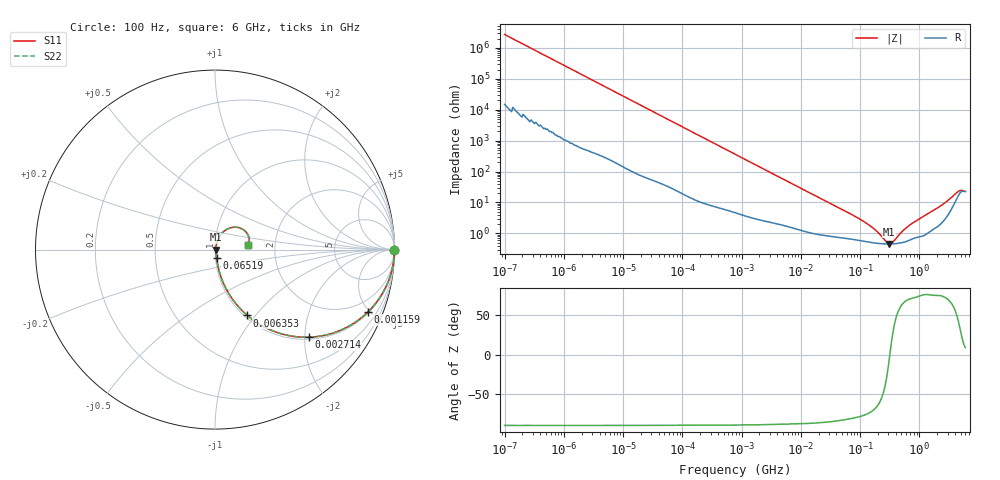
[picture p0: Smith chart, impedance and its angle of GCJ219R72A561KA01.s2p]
!Murata Part Number: GCJ219R72A561KA01
!These Parameters are Measured in Series Mode Connection
!Data Generated on Mar 13, 2026
!  o--ll--o
!Port1  Port2
!  o------o
!Operation Temp=25[degC], DC Bias Voltage=0[V]
!Freq. Start=100[Hz] Stop=6[GHz] 401[Steps]
# Hz S RI R 50
!Freq.(Hz) S11(Real) S11(Imag) S21(Real) S21(Imag) S12(Real) S12(Imag) S22(Real) S22(Imag)
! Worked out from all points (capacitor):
!   401 points, 100 Hz to 6 GHz, reference 50 ohm
!   read as one part in series: C = 580 pF near 109 Hz
!   lowest |Z| = 456 mohm at 312.4 MHz (marker M1)
!   series resonance near 318.1 MHz, so ESL is about 430 pH
!   S11 on the Smith chart (normalised r, x): 100 Hz: open; 1.159 MHz: 1.07, -4.88; 2.714 MHz: 1.05, -2.10; 6.353 MHz: 1.03, -0.91; 65.19 MHz: 1.01, -0.09; 6 GHz: 1.45, +0.07
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100  1 -3.65e-05  2e-07 3.65e-05  2e-07 3.65e-05  1 -3.65e-05
280  1 -0.000102  5e-07 0.000102  5e-07 0.000102  1 -0.000102
2008  1 -0.000728  3.5e-06 0.000728  3.5e-06 0.000728  1 -0.000728
40335  0.9997 -0.0145  0.0003 0.0145  0.0003 0.0145  0.9997 -0.0145
231233  0.9926 -0.0818  0.00737 0.0818  0.00737 0.0818  0.9926 -0.0818
774597  0.9272 -0.2535  0.0728 0.2535  0.0728 0.2535  0.9272 -0.2535
1159002  0.8528 -0.347  0.1472 0.347  0.1472 0.347  0.8528 -0.347
2713602  0.524 -0.4882  0.476 0.4882  0.476 0.4882  0.524 -0.4882
3882480  0.3561 -0.4651  0.6439 0.4651  0.6439 0.4651  0.3561 -0.4651
6353432  0.1797 -0.3666  0.8203 0.3666  0.8203 0.3666  0.1797 -0.3666
1.555665e7  0.043 -0.178  0.957 0.178  0.957 0.178  0.043 -0.178
6.518806e7  0.00859 -0.0441  0.9914 0.0441  0.9914 0.0441  0.00859 -0.0441
1.526266e8  0.00527 -0.0159  0.9947 0.0159  0.9947 0.0159  0.00527 -0.0159
1.996653e8  0.0048 -0.00965  0.9952 0.00965  0.9952 0.00965  0.0048 -0.00965
2.731619e8  0.00455 -0.00308  0.9955 0.00308  0.9955 0.00308  0.00455 -0.00308
3.124326e8  0.00453 -0.00036  0.9955 0.00036  0.9955 0.00036  0.00453 -0.00036
3.573489e8  0.00457 0.00238  0.9954 -0.00238  0.9954 -0.00238  0.00457 0.00238
5.346885e8  0.0052 0.0111  0.9948 -0.0111  0.9948 -0.0111  0.0052 0.0111
7.650043e8  0.00696 0.02  0.993 -0.02  0.993 -0.02  0.00696 0.02
2.562649e9  0.0314 0.0821  0.9686 -0.0821  0.9686 -0.0821  0.0314 0.0821
4.385646e9  0.1426 0.1192  0.8574 -0.1192  0.8574 -0.1192  0.1426 0.1192
6e9  0.1846 0.0242  0.8154 -0.0242  0.8154 -0.0242  0.1846 0.0242
